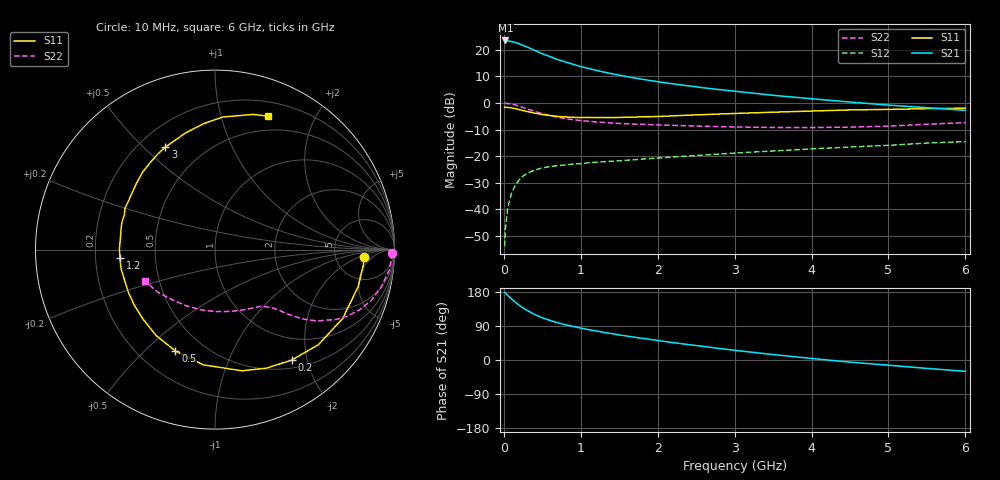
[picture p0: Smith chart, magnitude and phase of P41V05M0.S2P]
! SIEMENS Small Signal Semiconductors
! BFP182
! Si NPN RF Bipolar Junction Transistor in SOT143
! VCE = 1 V  IC = 5 mA
! Common Emitter S-Parameters:  March  1996
# GHz  S  MA  R  50
!  f  S11  S21  S12  S22
! GHz  MAG  ANG  MAG  ANG  MAG  ANG  MAG  ANG
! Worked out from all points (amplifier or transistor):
!   36 points, 10 MHz to 6 GHz, reference 50 ohm
!   highest |S21| = 23.6 dB at 20 MHz (marker M1)
!   |S21| within 3 dB of that: start of sweep to 344 MHz
!   unconditionally stable (mu >= 1): 1.455 GHz to end of sweep
!   at 250 MHz: K = 0.23, MSG = 24.6 dB, |S12| = -27.5 dB
!   at 1.4 GHz: K = 0.97, MSG = 16.5 dB, |S12| = -21.9 dB
!   at 6 GHz: K = 1.02, MAG = 4.9 dB, |S12| = -14.6 dB
!   S11 on the Smith chart (normalised r, x): 10 MHz: 10, -3; 200 MHz: 0.62, -1.74; 500 MHz: 0.35, -0.62; 1.2 GHz: 0.31, -0.04; 3 GHz: 0.31, +0.58; 6 GHz: 0.34, +1.41
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0.01  0.8325 -2.9  14.91 178.3  0.002 83.7  0.9877 -1.2
0.02  0.8307 -6.1  15.11 176.7  0.0042 88.0  0.9836 -2.5
0.05  0.8242 -14.5  14.92 170.5  0.0105 83.8  0.9796 -6.4
0.1  0.8082 -28.4  14.37 161.3  0.0198 74.7  0.9509 -12.4
0.15  0.7824 -42.6  13.83 152.4  0.0285 68.3  0.9158 -18.0
0.2  0.7495 -55.2  13.06 144.4  0.0359 62.3  0.8715 -22.7
0.25  0.7201 -66.5  12.2 137.2  0.042 56.9  0.8239 -26.8
0.3  0.6919 -77.4  11.43 131.2  0.0471 52.8  0.7761 -30.1
0.4  0.6455 -95.9  9.827 120.1  0.0544 45.6  0.6934 -35.0
0.5  0.6065 -111.3  8.478 111.5  0.0597 40.8  0.6301 -38.0
0.6  0.5805 -124.4  7.5 104.4  0.0632 37.8  0.5782 -40.1
0.7  0.5577 -135.8  6.585 98.4  0.0659 35.5  0.5384 -41.7
0.8  0.5463 -145.3  5.944 93.0  0.068 34.0  0.508 -42.8
1.1  0.5341 -168.6  4.483 80.1  0.0746 31.3  0.452 -45.8
1.2  0.5319 -174.8  4.13 76.6  0.0765 30.7  0.44 -46.9
1.7  0.54 159.4  2.957 60.1  0.0855 30.5  0.3996 -52.7
2.2  0.5719 140.1  2.292 45.9  0.0958 29.9  0.3792 -60.6
3  0.6348 115.8  1.671 25.6  0.1138 27.6  0.3536 -77.1
3.5  0.671 104.0  1.398 14.3  0.1247 25.5  0.3456 -89.5
4.5  0.7401 86.6  1.043 -5.7  0.1481 20.4  0.3513 -116.7
5.5  0.7824 74.3  0.817 -22.2  0.176 14.7  0.3978 -143.3
6  0.7993 68.5  0.726 -29.9  0.1871 10.3  0.4275 -155.7
